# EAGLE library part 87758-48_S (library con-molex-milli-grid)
HEADER
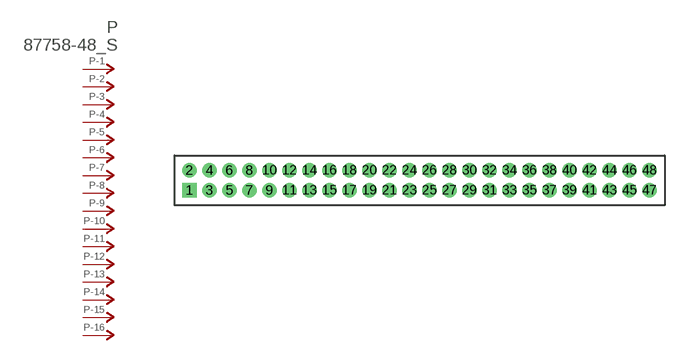
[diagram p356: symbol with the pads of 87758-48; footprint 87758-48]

Designator prefix P; gates -1=P-NV -2=P-N -3=P-N -4=P-N -5=P-N -6=P-N -7=P-N -8=P-N -9=P-N -10=P-N -11=P-N -12=P-N -13=P-N -14=P-N -15=P-N -16=P-N -17=P-N -18=P-N -19=P-N -20=P-N -21=P-N -22=P-N -23=P-N -24=P-N -25=P-N -26=P-N -27=P-N -28=P-N -29=P-N -30=P-N -31=P-N -32=P-N -33=P-N -34=P-N -35=P-N -36=P-N -37=P-N -38=P-N -39=P-N -40=P-N -41=P-N -42=P-N -43=P-N -44=P-N -45=P-N -46=P-N -47=P-N -48=P-N

## 87758-48_S  [87758-48]
1  -1:P  pas
2  -2:P  pas
3  -3:P  pas
4  -4:P  pas
5  -5:P  pas
6  -6:P  pas
7  -7:P  pas
8  -8:P  pas
9  -9:P  pas
10  -10:P  pas
11  -11:P  pas
12  -12:P  pas
13  -13:P  pas
14  -14:P  pas
15  -15:P  pas
16  -16:P  pas
17  -17:P  pas
18  -18:P  pas
19  -19:P  pas
20  -20:P  pas
21  -21:P  pas
22  -22:P  pas
23  -23:P  pas
24  -24:P  pas
25  -25:P  pas
26  -26:P  pas
27  -27:P  pas
28  -28:P  pas
29  -29:P  pas
30  -30:P  pas
31  -31:P  pas
32  -32:P  pas
33  -33:P  pas
34  -34:P  pas
35  -35:P  pas
36  -36:P  pas
37  -37:P  pas
38  -38:P  pas
39  -39:P  pas
40  -40:P  pas
41  -41:P  pas
42  -42:P  pas
43  -43:P  pas
44  -44:P  pas
45  -45:P  pas
46  -46:P  pas
47  -47:P  pas
48  -48:P  pas

## Footprint 87758-48 (pad centres in mm)
HEADER Dual Row, Vertical
drill 0.914 square: 1 -23,-1
drill 0.914: 2 -23,1; 3 -21,-1; 4 -21,1; 5 -19,-1; 6 -19,1; 7 -17,-1; 8 -17,1; 9 -15,-1; 10 -15,1; 11 -13,-1; 12 -13,1; 13 -11,-1; 14 -11,1; 15 -9,-1; 16 -9,1; 17 -7,-1; 18 -7,1; 19 -5,-1; 20 -5,1; 21 -3,-1; 22 -3,1; 23 -1,-1; 24 -1,1; 25 1,-1; 26 1,1; 27 3,-1; 28 3,1; 29 5,-1; 30 5,1; 31 7,-1; 32 7,1; 33 9,-1; 34 9,1; 35 11,-1; 36 11,1; 37 13,-1; 38 13,1; 39 15,-1; 40 15,1; 41 17,-1; 42 17,1; 43 19,-1; 44 19,1; 45 21,-1; 46 21,1; 47 23,-1; 48 23,1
